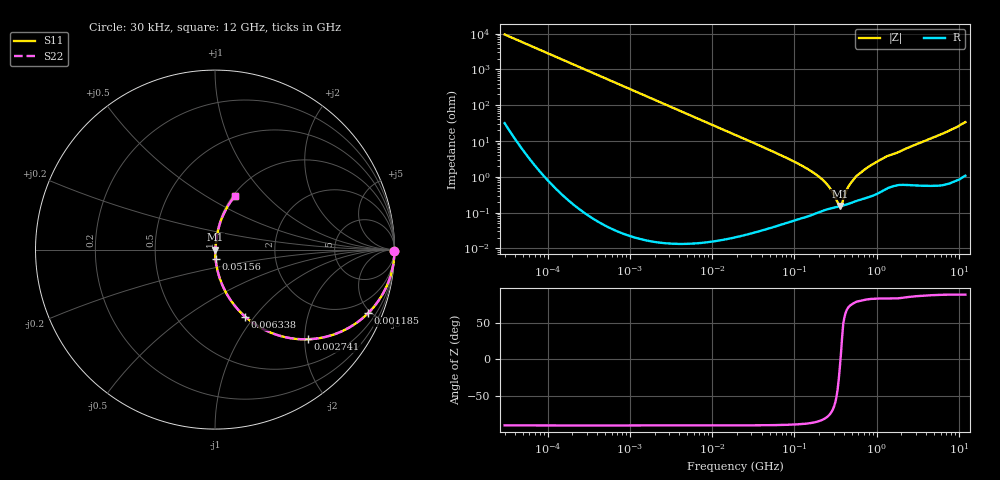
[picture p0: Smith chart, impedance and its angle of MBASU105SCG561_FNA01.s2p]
! MBASU105SCG561_FNA01  S-PARAMETER MODEL  ( General Type )
! Model Generated by TAIYO YUDEN Corporation (http://www.ty-top.com)
! Version 1.0
! TAIYO YUDEN Control No. 130207
! Copyright(c) 2013 TAIYO YUDEN CO.,LTD. All Rights Reserved.
! Product Description (link to TY-COMPAS)
! https://ds.yuden.co.jp/TYCOMPAS/or/detail?pn=MBASU105SCG561JFNA01&u=M
! Products Name : Multilayer Ceramic Capacitors
! Characteristics :
!  Capacitance : 560 pF , Rated Voltage : 50V , TCC : CG / C0G
!  Case Size : 1.0 x 0.5 / 0.039 x 0.02 [mm/inch] , Thickness : 0.5 / 0.02 [mm/inch]
!  (Conditions: Temperature = 25 degC , DC Bias Current/Voltage = 0A / 0V)
! External Node Assignments :
!  1  o---| |---o  2
! GND o---------o GND
! Frequency Range : 30000Hz  -  12GHz  [ 401 STEP ]
# MHz S RI R 50
! Freq[MHz].  S11 Real  S11 Imag  S21 Real  S21 Imag  S12 Real  S12 Imag  S22 Real  S22 Imag
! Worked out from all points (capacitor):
!   401 points, 30 kHz to 12 GHz, reference 50 ohm
!   read as one part in series: C = 558 pF near 32 kHz
!   lowest |Z| = 152 mohm at 357 MHz (marker M1)
!   series resonance near 363.6 MHz, so ESL is about 340 pH
!   S11 on the Smith chart (normalised r, x): 30 kHz: open; 1.185 MHz: 1.00, -4.81; 2.741 MHz: 1.00, -2.08; 6.338 MHz: 1.00, -0.90; 51.56 MHz: 1.00, -0.11; 12 GHz: 1.02, +0.68
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0.03  0.9999 -0.0105  0.000146 0.0105  0.000146 0.0105  0.9999 -0.0105
0.260295  0.9917 -0.0905  0.00827 0.0905  0.00827 0.0905  0.9917 -0.0905
0.642112  0.9517 -0.2143  0.0483 0.2143  0.0483 0.2143  0.9517 -0.2143
1.184973  0.8527 -0.3543  0.1473 0.3543  0.1473 0.3543  0.8527 -0.3543
2.258455  0.6145 -0.4867  0.3855 0.4867  0.3855 0.4867  0.6145 -0.4867
2.740579  0.5198 -0.4995  0.4802 0.4995  0.4802 0.4995  0.5198 -0.4995
6.338349  0.1683 -0.374  0.8317 0.374  0.8317 0.374  0.1683 -0.374
10.28143  0.0714 -0.2573  0.9286 0.2573  0.9286 0.2573  0.0714 -0.2573
18.97367  0.0222 -0.1465  0.9778 0.1465  0.9778 0.1465  0.0222 -0.1465
51.55976  0.0033 -0.054  0.9967 0.054  0.9967 0.054  0.0033 -0.054
164.6252  0.00105 -0.0137  0.9989 0.0137  0.9989 0.0137  0.00105 -0.0137
250.359  0.00126 -0.00597  0.9987 0.00597  0.9987 0.00597  0.00126 -0.00597
284.8288  0.00134 -0.00385  0.9987 0.00385  0.9987 0.00385  0.00134 -0.00385
334.6645  0.00144 -0.00129  0.9986 0.00129  0.9986 0.00129  0.00144 -0.00129
356.9603  0.00149 -0.000291  0.9985 0.000291  0.9985 0.000291  0.00149 -0.000291
380.7415  0.00155 0.000909  0.9985 -0.000909  0.9985 -0.000909  0.00155 0.000909
462.0203  0.0018 0.00542  0.9982 -0.00542  0.9982 -0.00542  0.0018 0.00542
560.6502  0.00218 0.0099  0.9978 -0.0099  0.9978 -0.0099  0.00218 0.0099
799.3715  0.00304 0.0189  0.997 -0.0189  0.997 -0.0189  0.00304 0.0189
1428.372  0.00654 0.039  0.9935 -0.039  0.9935 -0.039  0.00654 0.039
5188.566  0.0226 0.1292  0.9774 -0.1292  0.9774 -0.1292  0.0226 0.1292
12000  0.1099 0.2973  0.8901 -0.2973  0.8901 -0.2973  0.1099 0.2973
